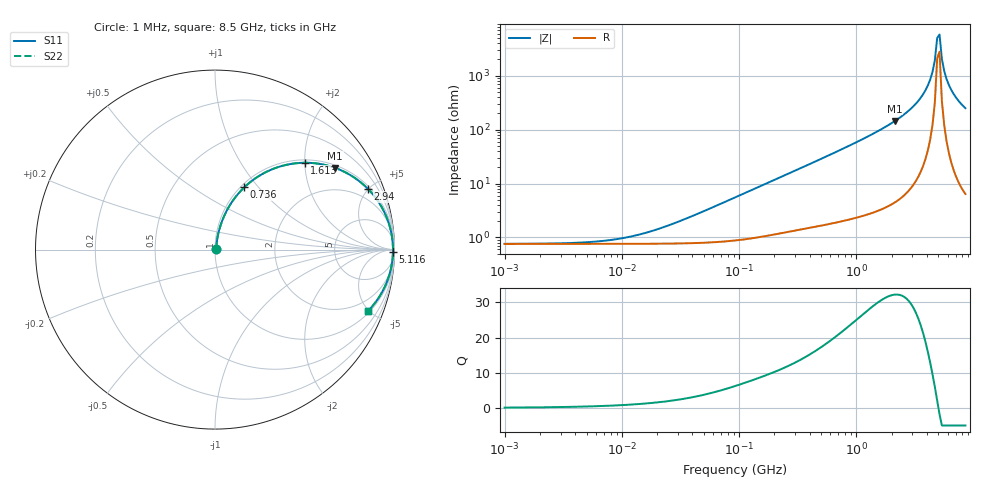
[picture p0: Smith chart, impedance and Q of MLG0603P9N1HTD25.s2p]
! S-Parameter Data Generated by TDK Corporation
! Copyright(C) 2025 TDK Corporation.
! All Rights Reserved.
! TDK P/N: MLG0603P9N1HTD25 (SMD / SMT Inductor (Coil))
! Property: L=9.1nH at 500MHz
! Size(LxWxT): 0.6x0.3x0.3mm
! Model Type: s2p (Touchstone File Format Version 1.0)
! Frequency: DC=Yes Start=1MHz Stop=8500MHz 198points Log-sweep
! Model Generated on Feb. 6, 2025
! Terms and conditions regarding TDK Simulation Models:
! 1)This simulation model is being provided solely for informational
!  purposes. Please refer to the specifications of the products in
!  terms of detailed characteristics of such products.
! 2)In no event shall TDK Corporation of any of its subsidiaries be
!  liable for any loss or damage arising, directly or indirectly,
!  from any information contained in this simulation model, including,
!  but not limited to loss or damages arising from any inaccuracies,
!  omissions or errors in connection with such information.
! 3)Any and all copyrights on this simulation model are owned by
!  TDK Corporation.  Duplication or redistribution of this simulation
!  model without prior written permission from TDK Corporation
!  is prohibited.
! 4)This simulation model is subject to any modification or change
!  without any prior notice.
! 5)Neither TDK Corporation nor any of its subsidiaries shall make any
!  warranty, express or implied, including but not limited to the
!  correctness, implied warranties of merchantability and fitness for
!  a particular purpose with respect to this simulation models.
! 6)The use of this simulation model shall be deemed to have consented
!  to the terms and conditions hereof.
! Port Assignments:
!  1 ---@@@--- 2
! Applicable Conditions:
!  Temperature = 25 degC
!  DC Bias Current = 0 A
!  Small Signal Operation
# Hz S MA R 50
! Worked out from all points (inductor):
!   197 points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, 1 MHz to 8.5 GHz, reference 50 ohm
!   read as one part in series: L = 9.46 nH near 40.16 MHz
!   highest Q = 32.2 at 2.128 GHz (marker M1), where L = 10.8 nH
!   self-resonance near 4.885 GHz
!   S11 on the Smith chart (normalised r, x): 1 MHz: 1.02, +0.00; 736 MHz: 1.04, +0.85; 1.613 GHz: 1.07, +2.00; 2.94 GHz: 1.17, +4.95; 5.116 GHz: open; 8.5 GHz: 1.13, -4.98
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1000000  0.007566 4.4  0.9925 -0.0  0.9925 -0.0  0.007566 4.4
4587603  0.008019 19.6  0.9925 -0.2  0.9925 -0.2  0.008019 19.6
1.005548e7  0.009617 37.8  0.9924 -0.3  0.9924 -0.3  0.009617 37.8
2.10461e7  0.01458 57.8  0.9923 -0.7  0.9923 -0.7  0.01458 57.8
9.219544e7  0.05462 77.7  0.9898 -3.1  0.9898 -3.1  0.05462 77.7
4.229561e8  0.2324 72.9  0.9579 -13.4  0.9579 -13.4  0.2324 72.9
7.359901e8  0.3832 64.8  0.9059 -22.5  0.9059 -22.5  0.3832 64.8
1.613203e9  0.6959 44.1  0.6957 -44.1  0.6957 -44.1  0.6959 44.1
1.940355e9  0.773 37.6  0.6106 -50.6  0.6106 -50.6  0.773 37.6
2.128028e9  0.8094 34.2  0.5626 -54.0  0.5626 -54.0  0.8094 34.2
2.939772e9  0.9166 21.7  0.37 -66.4  0.37 -66.4  0.9166 21.7
3.703002e9  0.9666 12.4  0.2147 -74.9  0.2147 -74.9  0.9666 12.4
4.253027e9  0.9841 6.7  0.1175 -78.9  0.1175 -78.9  0.9841 6.7
4.453958e9  0.9877 4.8  0.08469 -79.2  0.08469 -79.2  0.9877 4.8
4.664383e9  0.9901 2.9  0.05192 -77.6  0.05192 -77.6  0.9901 2.9
4.884749e9  0.9915 1.0  0.01994 -64.2  0.01994 -64.2  0.9915 1.0
5.115526e9  0.9917 -0.9  0.01716 60.5  0.01716 60.5  0.9917 -0.9
5.357206e9  0.9907 -2.8  0.0489 77.7  0.0489 77.7  0.9907 -2.8
5.610304e9  0.9886 -4.7  0.08173 79.7  0.08173 79.7  0.9886 -4.7
5.87536e9  0.9854 -6.6  0.1146 79.4  0.1146 79.4  0.9854 -6.6
6.748056e9  0.9689 -12.3  0.2126 75.5  0.2126 75.5  0.9689 -12.3
8.5e9  0.9197 -21.7  0.3696 66.8  0.3696 66.8  0.9197 -21.7
